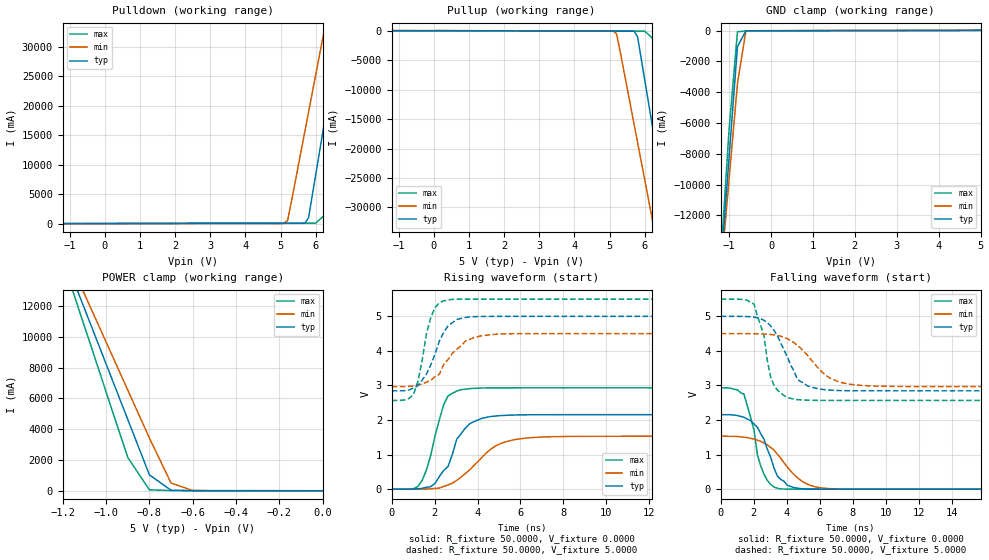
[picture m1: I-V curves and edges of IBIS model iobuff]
| IBIS file iobuff.ibs created by s2ibis2 version 1.1
| North Carolina State University Electronics Research Laboratory  1995
[IBIS ver]   2.1
[File name]   iobuff.ibs
[File Rev]   0.1
[Date]   Sep 29, 1999
[Source]   Spice simulations on CADENCE spice models
[Notes]   This Model was done by Pradeep Mishra
[Disclaimer]   This is for modelling purposes only.Accuracy is not guaranteed
[Copyright]   CADENCE DESIGN SYSTEMS INC
|   Component Component-Name
[Component]   Component-Name
[Manufacturer]   Manufacturer-Name
[Package]
| variable   typ   min   max
R_pkg   0.0000   0.0000   0.0000
L_pkg   0.0000H   0.0000H   0.0000H
C_pkg   0.0000F   0.0000F   0.0000F
[Pin]  signal_name   model_name   R_pin   L_pin   C_pin
pad   pad   iobuff
| inputinput   none
| ena  ena   none
vdd   vdd   POWER
vss   vss   GND
| Models and submodels in the file (1): iobuff (I/O)
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|   Model iobuff
[Model]   iobuff
Model_type   I/O
Polarity   Inverting
Enable   Active-High
Vinl =   0.8000V
Vinh =   2.0000V
Vmeas =   1.5000V
Cref =  10.0000pF
Rref =  55.0000
Vref =   2.5000V
C_comp   5.0000pF   5.0000pF   5.0000pF
[Temperature Range]   50.0000   100.0000   0.0000
[Voltage Range]   5.0000V   4.5000V   5.5000V
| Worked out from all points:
|   slope of the pulldown table from 0 to 0.75 V, typ, clamps not added: 101 ohm
|   slope of the pullup table from 0 to 0.75 V, typ, clamps not added: 2.28 kohm
|   rising waveform, R_fixture 50.0000, V_fixture 0.0000: 20-80 % time 1.09ns typ, 1.64ns min, 743ps max; typ from 0 V to 2.15 V
|   rising waveform, R_fixture 50.0000, V_fixture 5.0000: 20-80 % time 904ps typ, 1.23ns min, 569ps max; typ from 2.85 V to 5 V
|   falling waveform, R_fixture 50.0000, V_fixture 0.0000: 20-80 % time 1.09ns typ, 1.74ns min, 847ps max; typ from 2.15 V to 0 V
|   falling waveform, R_fixture 50.0000, V_fixture 5.0000: 20-80 % time 1.3ns typ, 1.87ns min, 812ps max; typ from 5 V to 2.85 V
[Pulldown]
| voltage   I(typ)   I(min)   I(max)
-5V       -40.06mA   -30.13mA   -54.39mA
5.1V      55.2mA     58.89mA    85.46mA
5.2V      55.36mA    536.5mA    85.82mA
5.3V      55.56mA    3.453A     86.12mA
5.7V      85.01mA    15.89A     86.96mA
5.8V      1.081A     19.01A     87.24mA
6V        8.264A     25.23A     87.97mA
6.4V      22.63A     37.67A     2.226A
6.8V      37A        50.11A     19.22A
7.2V      51.37A     62.56A     36.22A
10V       152A       149.7A     155.2A
[Pullup]
| voltage   I(typ)   I(min)   I(max)
-5V       40.06mA    30.23mA    54.38mA
5.1V      -55.2mA    -58.89mA   -85.46mA
5.2V      -55.36mA   -536.5mA   -85.82mA
5.3V      -55.56mA   -3.453A    -86.12mA
5.7V      -85.01mA   -15.89A    -86.96mA
5.8V      -1.081A    -19.01A    -87.24mA
6V        -8.264A    -25.23A    -87.97mA
6.4V      -22.63A    -37.67A    -2.226A
6.8V      -37A       -50.11A    -19.22A
7.2V      -51.37A    -62.56A    -36.22A
10V       -152A      -149.7A    -155.2A
[GND_clamp]
| voltage   I(typ)   I(min)   I(max)
-5V       -152A      -134.1A    -176.5A
-1.2V     -15.42A    -15.88A    -14.92A
-1V       -8.232A    -9.654A    -6.423A
-800mV    -1.047A    -3.432A    -79.61mA
-600mV    -21.51mA   -36.29mA   -31.42mA
5V        13.77mA    14.06mA    14.93mA
[POWER_clamp]
| voltage   I(typ)   I(min)   I(max)
-5V       152A       134.1A     176.5A
-1.2V     15.42A     15.88A     14.92A
-1.1V     11.82A     12.77A     10.67A
-1V       8.232A     9.654A     6.423A
-900mV    4.64A      6.543A     2.173A
-800mV    1.047A     3.432A     79.61mA
-700mV    50.28mA    514.6mA    33.89mA
-600mV    21.51mA    36.29mA    31.42mA
0V        13.77mA    8.907mA    21.63mA
[Ramp]
| variable   typ   min   max
dV/dt_r   1.2928/1.0519n   0.9186/1.5798n   1.7598/0.6641n
dV/dt_f   1.2928/1.2529n   0.9186/1.8472n   1.7598/0.8063n
R_load = 50.0000
[Rising Waveform]
R_fixture = 50.0000
V_fixture = 0.0000
| time   V(typ)   V(min)   V(max)
0s        258.3pV    5.342nV    226.8pV
1.01ns    3.428mV    134.9uV    10.98mV
1.414ns   24.71mV    1.828mV    249.7mV
2.02ns    168.5mV    21.99mV    1.542V
2.424ns   541.4mV    78.77mV    2.45V
3.232ns   1.604V     348.3mV    2.879V
3.838ns   1.957V     690.8mV    2.916V
4.848ns   2.116V     1.255V     2.931V
6.263ns   2.151V     1.477V     2.933V
20ns      2.155V     1.531V     2.933V
[Rising Waveform]
R_fixture = 50.0000
V_fixture = 5.0000
V_fixture_min = 4.5000
V_fixture_max = 5.5000
| time   V(typ)   V(min)   V(max)
0s        2.845V     2.969V     2.567V
1.01ns    2.928V     2.986V     2.737V
1.212ns   2.99V      3.012V     3.097V
1.616ns   3.327V     3.096V     4.492V
1.818ns   3.589V     3.15V      4.957V
2.02ns    3.913V     3.255V     5.258V
2.424ns   4.534V     3.608V     5.448V
3.434ns   4.968V     4.284V     5.499V
4.848ns   4.999V     4.481V     5.5V
20ns      5V         4.5V       5.5V
[Falling Waveform]
R_fixture = 50.0000
V_fixture = 0.0000
| time   V(typ)   V(min)   V(max)
0s        2.155V     1.531V     2.933V
1.414ns   2.08V      1.503V     2.747V
2.02ns    1.882V     1.45V      1.698V
2.222ns   1.794V     1.417V     1.002V
2.424ns   1.606V     1.385V     675mV
2.828ns   1.153V     1.284V     252.3mV
3.434ns   381.1mV    1.009V     24.2mV
4.848ns   15.51mV    256.4mV    88.08uV
6.061ns   543.5uV    39.13mV    838.1nV
20ns      -144.8nV   -546.8nV   -1.547uV
[Falling Waveform]
R_fixture = 50.0000
V_fixture = 5.0000
V_fixture_min = 4.5000
V_fixture_max = 5.5000
| time   V(typ)   V(min)   V(max)
0s        5V         4.5V       5.5V
2.02ns    4.977V     4.498V     5.356V
2.626ns   4.883V     4.489V     4.434V
3.03ns    4.723V     4.474V     3.243V
4.242ns   3.593V     4.295V     2.625V
4.646ns   3.182V     4.156V     2.591V
5.253ns   2.989V     3.881V     2.574V
6.465ns   2.872V     3.263V     2.567V
7.677ns   2.849V     3.05V      2.567V
20ns      2.845V     2.969V     2.567V
